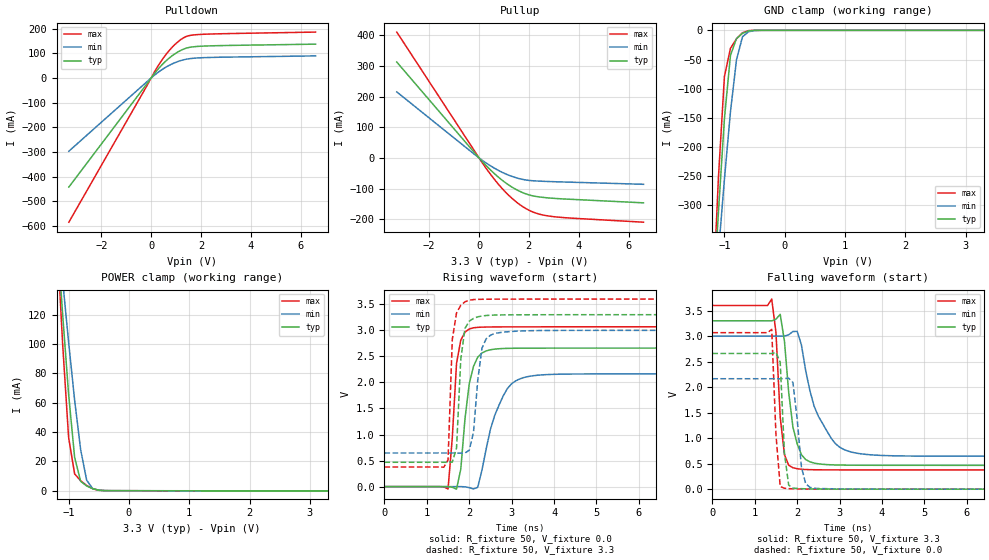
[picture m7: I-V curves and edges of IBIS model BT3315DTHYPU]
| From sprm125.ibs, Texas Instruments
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[Model]   BT3315DTHYPU
Model_type   I/O
Vinh = 2.00
Vinl = 0.80
Enable   Active-Low
Polarity   Non-Inverting
| signals   A, GZ, Y
Vmeas = 1.5
|   typ   min   max
C_comp   1.5797p   1.5046p   1.7659p
|   typ   min   max
[Temperature Range]   25   -40   125
|   typ   min   max
[Voltage Range]   3.30V   3.00V   3.60V
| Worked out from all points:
|   slope of the pulldown table from 0 to 0.495 V, typ, clamps not added: 8.32 ohm
|   slope of the pullup table from 0 to 0.495 V, typ, clamps not added: 11.7 ohm
|   GND clamp passes 1 mA (typ) near -0.60 V on its own axis
|   POWER clamp passes 1 mA (typ) near -0.56 V on its own axis
|   rising waveform, R_fixture 50, V_fixture 0.0: 20-80 % time 225ps typ, 467ps min, 153ps max; typ from 0 V to 2.66 V
|   falling waveform, R_fixture 50, V_fixture 3.3: 20-80 % time 239ps typ, 557ps min, 146ps max; typ from 3.3 V to 0.467 V
|   rising waveform, R_fixture 50, V_fixture 3.3: 20-80 % time 131ps typ, 172ps min, 104ps max; typ from 0.467 V to 3.3 V
|   falling waveform, R_fixture 50, V_fixture 0.0: 20-80 % time 107ps typ, 151ps min, 112ps max; typ from 2.66 V to 0 V
[Pulldown]
|   Voltage   I(typ)   I(min)   I(max)
-3.3V     -442.4mA   -297mA     -585.1mA
200mV     26.32mA    16.85mA    36.03mA
600mV     69.7mA     44.45mA    95.88mA
800mV     86.89mA    55.25mA    119.9mA
1.1V      107.2mA    67.8mA     148.9mA
1.4V      120.9mA    76.03mA    168.1mA
1.9V      128.4mA    81.62mA    176.5mA
6.6V      137.5mA    89.79mA    186.4mA
[GND_clamp]
|   Voltage   I(typ)   I(min)   I(max)
-3.3V     -4.679A    -3.53A     -6.074A
-1.2V     -491.5mA   -514.1mA   -484.3mA
-1.1V     -312.5mA   -381.7mA   -253.3mA
-1V       -151.4mA   -255.1mA   -79.17mA
-900mV    -42.95mA   -139.8mA   -30.75mA
-800mV    -14.03mA   -50.51mA   -14.62mA
-700mV    -5.033mA   -10.94mA   -4.188mA
-600mV    -961.3uA   -2.448mA   -466.6uA
-400mV    -4.855uA   -52.49uA   -479.3nA
3.3V      222pA      4.204uA    44.41pA
[Pullup]
|   Voltage   I(typ)   I(min)   I(max)
-3.3V     312.8mA    215.3mA    410.6mA
-200mV    18.7mA     12.62mA    24.95mA
300mV     -26.42mA   -17.41mA   -35.83mA
900mV     -71.08mA   -45.91mA   -97.39mA
1.2V      -88.97mA   -56.76mA   -122.7mA
1.5V      -103.7mA   -65.18mA   -144.2mA
1.8V      -115mA     -71.04mA   -161.5mA
2.1V      -122.8mA   -74.28mA   -174.6mA
2.7V      -130.1mA   -76.86mA   -188.5mA
3.6V      -134.9mA   -79.17mA   -196.2mA
6.6V      -146.8mA   -86.25mA   -209.9mA
[POWER_clamp]
|   Voltage   I(typ)   I(min)   I(max)
-3.3V     1.566A     1.185A     2.029A
-1.2V     180.9mA    188mA      178.7mA
-1.1V     121.1mA    143.9mA    100.9mA
-1V       65.87mA    101.4mA    36.44mA
-900mV    22.73mA    61.78mA    11.46mA
-800mV    6.428mA    27.98mA    6.813mA
-700mV    3.2mA      7.12mA     3.57mA
-600mV    1.373mA    1.452mA    1.296mA
-500mV    357.3uA    341.4uA    240.6uA
-400mV    65.6uA     67.61uA    56.84uA
3.3V      -108.3uA   -68.36uA   -162.1uA
[Ramp]
|   I(typ)   I(min)   I(max)
dV/dt_r   1.596/0.219n   1.299/0.467n   1.840/0.133n
dV/dt_f   1.700/0.234n   1.413/0.559n   1.934/0.132n
[Rising Waveform]
R_fixture = 50
V_fixture = 0.0
|  pu_on
|  TIME   V(typ)   V(min)   V(max)
0s        1nV        11nV       1nV
1.5ns     1.188mV    119.5uV    -44.73mV
1.6ns     -12.6mV    280.8uV    938.5mV
1.7ns     -48.76mV   522.6uV    2.364V
1.8ns     333.9mV    940.3uV    2.811V
2ns       1.977V     -19.15mV   3.026V
2.3ns     2.565V     319.2mV    3.061V
2.6ns     2.639V     1.367V     3.065V
3.2ns     2.657V     2.07V      3.067V
10ns      2.659V     2.164V     3.067V
[Falling Waveform]
R_fixture = 50
V_fixture = 3.3
V_fixture_min = 3.0
V_fixture_max = 3.6
|  pd_on
|  TIME   V(typ)   V(min)   V(max)
0s        3.3V       3V         3.6V
1.4ns     3.298V     3V         3.726V
1.5ns     3.333V     3V         3.07V
1.6ns     3.427V     2.998V     1.415V
1.7ns     2.902V     3V         675.2mV
1.9ns     1.216V     3.09V      420.4mV
2.1ns     675.9mV    2.829V     390.3mV
2.5ns     496.8mV    1.429V     379.6mV
3.2ns     470.2mV    745.7mV    377.3mV
10ns      467.3mV    645.6mV    376.8mV
[Rising Waveform]
R_fixture = 50
V_fixture = 3.3
V_fixture_min = 3.0
V_fixture_max = 3.6
|  pd_off
|  TIME   V(typ)   V(min)   V(max)
0s        467.3mV    645.6mV    376.8mV
1.5ns     466.6mV    646mV      512.6mV
1.6ns     470.2mV    645.7mV    2.824V
1.7ns     740.1mV    644.8mV    3.335V
1.8ns     2.444V     642.6mV    3.479V
1.9ns     3.04V      644.5mV    3.547V
2.1ns     3.228V     1.041V     3.59V
2.3ns     3.275V     2.658V     3.596V
2.6ns     3.293V     2.94V      3.598V
10ns      3.3V       3V         3.6V
[Falling Waveform]
R_fixture = 50
V_fixture = 0.0
|  pu_off
|  TIME   V(typ)   V(min)   V(max)
0s        2.659V     2.164V     3.067V
1.4ns     2.658V     2.164V     3.131V
1.5ns     2.683V     2.163V     1.068V
1.6ns     2.486V     2.164V     51.29mV
1.7ns     700.6mV    2.167V     18.36mV
1.8ns     79.16mV    2.174V     10.34mV
1.9ns     21.47mV    2.091V     6.702mV
2.1ns     9.853mV    437.2mV    3.039mV
2.3ns     5.394mV    36.04mV    1.716mV
10ns      1.515uV    3.915uV    144nV
